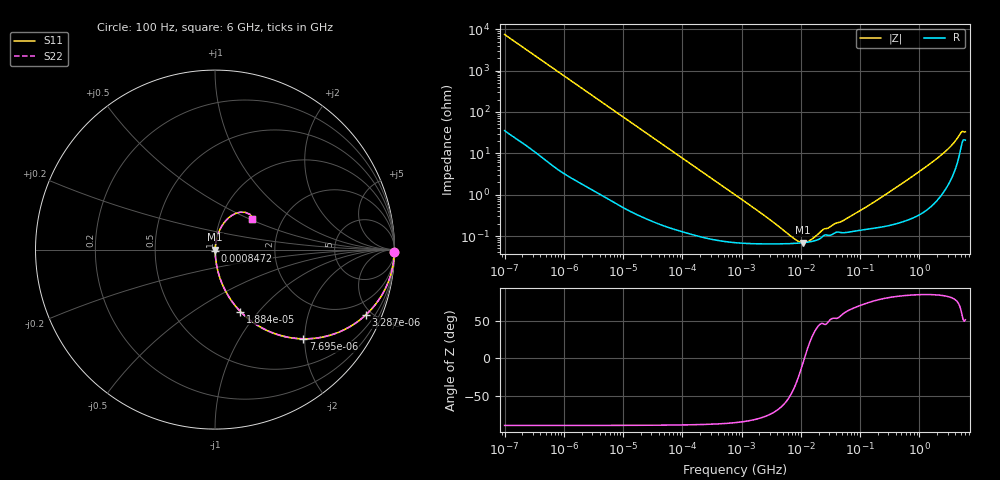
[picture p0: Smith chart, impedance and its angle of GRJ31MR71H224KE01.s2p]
!Murata Part Number: GRJ31MR71H224KE01
!These Parameters are Measured in Series Mode Connection
!Data Generated on Jun 19, 2026
!  o--ll--o
!Port1  Port2
!  o------o
!Operation Temp=25[degC], DC Bias Voltage=0[V]
!Freq. Start=100[Hz] Stop=6[GHz] 401[Steps]
# Hz S RI R 50
!Freq.(Hz) S11(Real) S11(Imag) S21(Real) S21(Imag) S12(Real) S12(Imag) S22(Real) S22(Imag)
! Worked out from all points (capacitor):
!   401 points, 100 Hz to 6 GHz, reference 50 ohm
!   read as one part in series: C = 212 nF near 109 Hz
!   lowest |Z| = 69.1 mohm at 10.87 MHz (marker M1)
!   series resonance near 11.5 MHz, so ESL is about 900 pH
!   S11 on the Smith chart (normalised r, x): 100 Hz: open; 3.287 kHz: 1.02, -4.60; 7.695 kHz: 1.01, -1.97; 18.84 kHz: 1.01, -0.81; 847.2 kHz: 1.00, -0.02; 6 GHz: 1.41, +0.52
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100  0.9998 -0.0134  0.000242 0.0134  0.000242 0.0134  0.9998 -0.0134
600  0.9933 -0.0792  0.00665 0.0792  0.00665 0.0792  0.9933 -0.0792
2008  0.9327 -0.2481  0.0673 0.2481  0.0673 0.2481  0.9327 -0.2481
3287  0.8395 -0.3644  0.1605 0.3644  0.1605 0.3644  0.8395 -0.3644
7695  0.4922 -0.4969  0.5078 0.4969  0.5078 0.4969  0.4922 -0.4969
12592  0.2678 -0.4394  0.7322 0.4394  0.7322 0.4394  0.2678 -0.4394
18841  0.1418 -0.345  0.8582 0.345  0.8582 0.345  0.1418 -0.345
40335  0.0362 -0.1817  0.9638 0.1817  0.9638 0.1817  0.0362 -0.1817
129199  0.00463 -0.059  0.9954 0.059  0.9954 0.059  0.00463 -0.059
774597  0.000788 -0.00994  0.9992 0.00994  0.9992 0.00994  0.000788 -0.00994
847162  0.000764 -0.00909  0.9992 0.00909  0.9992 0.00909  0.000764 -0.00909
7947587  0.000663 -0.000508  0.9993 0.000508  0.9993 0.000508  0.000663 -0.000508
1.087309e7  0.000687 -7.52e-05  0.9993 7.52e-05  0.9993 7.52e-05  0.000687 -7.52e-05
1.555665e7  0.000742 0.000412  0.9993 -0.000412  0.9993 -0.000412  0.000742 0.000412
2.434276e7  0.00102 0.00105  0.999 -0.00105  0.999 -0.00105  0.00102 0.00105
5.449875e7  0.00121 0.00214  0.9988 -0.00214  0.9988 -0.00214  0.00121 0.00214
3.124326e8  0.00192 0.0114  0.9981 -0.0114  0.9981 -0.0114  0.00192 0.0114
1.309207e9  0.00635 0.047  0.9936 -0.047  0.9936 -0.047  0.00635 0.047
2.931063e9  0.0285 0.1141  0.9715 -0.1141  0.9715 -0.1141  0.0285 0.1141
4.009986e9  0.0693 0.1706  0.9307 -0.1706  0.9307 -0.1706  0.0693 0.1706
4.796499e9  0.1388 0.2081  0.8612 -0.2081  0.8612 -0.2081  0.1388 0.2081
6e9  0.208 0.1698  0.792 -0.1698  0.792 -0.1698  0.208 0.1698
